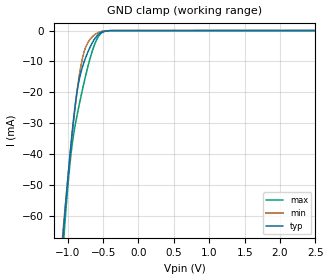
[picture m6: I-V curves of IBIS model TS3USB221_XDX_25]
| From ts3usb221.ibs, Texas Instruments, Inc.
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[Model]   TS3USB221_XDX_25
Model_type  Terminator
| variable   typ   min   max
C_comp   2.13pF   1.84pF   2.42pF
| C_tri-state   2.13pF   1.84pF   2.42pF
[Temperature Range]   40   100   -40
| Ambient temperature   25   85   -40
[Voltage range]   2.5   2.3   2.7
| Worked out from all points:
|   GND clamp passes 1 mA (typ) near -0.55 V on its own axis
[GND Clamp]
| TS3USB221_XDX_25
|   Voltage   I(typ)   I(min)   I(max)
-2.5V     -555mA     -505.6mA   -605.4mA
-1.07V    -67.94mA   -66.04mA   -72mA
-1.06V    -65.07mA   -63.46mA   -68.83mA
-1.045V   -60.82mA   -59.62mA   -64.18mA
-970mV    -40.79mA   -41.25mA   -43.58mA
-910mV    -27.17mA   -27.94mA   -32.74mA
-870mV    -20.14mA   -20.16mA   -27.72mA
-820mV    -14.17mA   -12.29mA   -22.14mA
-730mV    -7.817mA   -4.59mA    -13.07mA
-595mV    -1.951mA   -945.1uA   -3.15mA
-400mV    -32.2uA    -20.14uA   -24.65uA
2.5V      511.7pA    1.019nA    45.54pA
